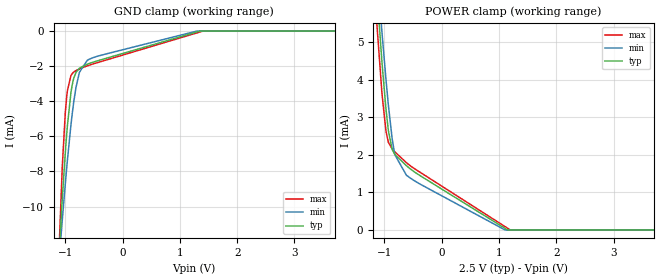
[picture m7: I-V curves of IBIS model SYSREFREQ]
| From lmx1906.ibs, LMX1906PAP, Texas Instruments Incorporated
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|   Model SYSREFREQ
[Model]   SYSREFREQ
Model_type   Input
Vinl = 0.4
Vinh = 1.4
|   typ   min   max
C_comp   0.266pF   0.263pF   0.269pF
[Voltage Range]   2.5   2.4   2.6
[Temperature Range]   27   105   -40
[Power Clamp Reference]   2.5   2.4   2.6
[GND Clamp Reference]   0   0   0
[GND Clamp]
|   Voltage   I(typ)   I(min)   I(max)
-2.5V     -117.2mA   -84.14mA   -199mA
-1.113V   -12.98mA   -13.29mA   -12.82mA
-1.052V   -9.564mA   -10.78mA   -7.743mA
-1V       -6.949mA   -8.719mA   -4.665mA
-962.5mV  -5.379mA   -7.35mA    -3.391mA
-895mV    -3.376mA   -5.173mA   -2.501mA
-857.5mV  -2.75mA    -4.166mA   -2.347mA
-812.5mV  -2.349mA   -3.196mA   -2.25mA
-752.5mV  -2.113mA   -2.342mA   -2.157mA
-572.5mV  -1.835mA   -1.591mA   -1.931mA
1.4V      0A         0A         -3.341uA
5V        0A         0A         0A
[POWER Clamp]
|   Voltage   I(typ)   I(min)   I(max)
-2.5V     58.4mA     58.67mA    55.42mA
-1.427V   12.66mA    12.7mA     11.61mA
-1.045V   4.49mA     5.282mA    3.657mA
-977.5mV  3.282mA    4.071mA    2.682mA
-932.5mV  2.648mA    3.331mA    2.334mA
-865mV    2.141mA    2.418mA    2.154mA
-820mV    2.011mA    2.004mA    2.08mA
-617.5mV  1.711mA    1.458mA    1.791mA
-362.5mV  1.431mA    1.208mA    1.52mA
1.1V      46.27uA    3.927uA    94.01uA
1.205V    0A         0A         0A
5V        0A         0A         0A
